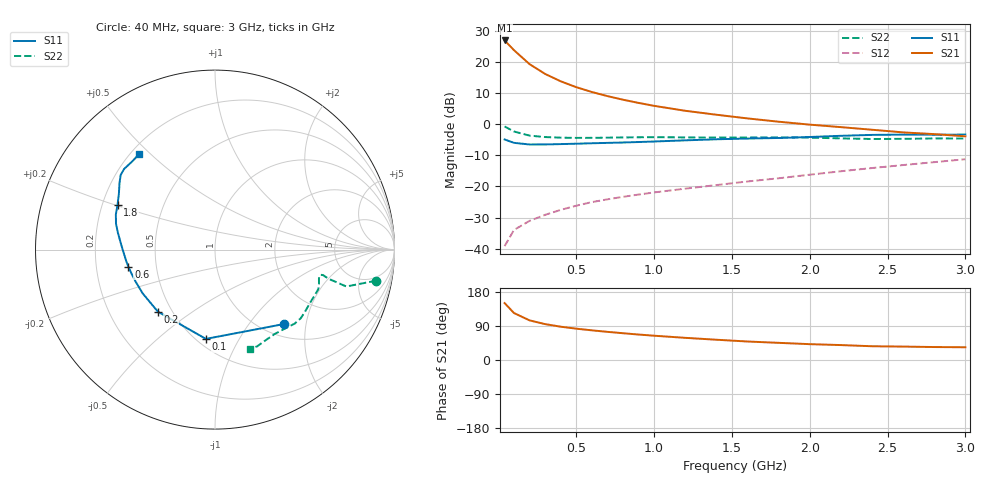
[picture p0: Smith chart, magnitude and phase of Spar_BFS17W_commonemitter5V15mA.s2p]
! Filename:  BFS17WD.S2P  Version:  4.0
! NXP part #: BFS17W  Date: Jun 1994
! Bias condition: Vce=5V, Ic=15mA
#  MHz  S  MA  R  50
! Freq  S11  S21  S12  S22  !GUM [dB]
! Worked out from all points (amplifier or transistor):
!   21 points, 40 MHz to 3 GHz, reference 50 ohm
!   highest |S21| = 26.8 dB at 40 MHz (marker M1)
!   |S21| within 3 dB of that: start of sweep to 97.95 MHz
!   unconditionally stable (mu >= 1): 325.1 MHz to 2.07 GHz
!   at 300 MHz: K = 0.98, MSG = 22.6 dB, |S12| = -29.1 dB
!   at 1 GHz: K = 1.20, MAG = 11.2 dB, |S12| = -21.9 dB
!   at 3 GHz: K = 0.95, MSG = 3.7 dB, |S12| = -11.3 dB
!   S11 on the Smith chart (normalised r, x): 40 MHz: 1.24, -1.51; 100 MHz: 0.56, -0.74; 200 MHz: 0.42, -0.37; 600 MHz: 0.34, -0.09; 1.8 GHz: 0.26, +0.21; 3 GHz: 0.23, +0.46
40  0.566 -47.1  21.93 150.2  0.011 71.1  0.915 -10.9
100  0.5 -95.8  15.33 124.0  0.02 58.8  0.76 -15.7
200  0.47 -132.6  9.156 104.6  0.028 57.9  0.653 -14.4
300  0.471 -148.7  6.371 94.7  0.035 59.9  0.619 -13.3
400  0.477 -158.0  4.854 87.9  0.042 62.8  0.605 -13.4
500  0.484 -164.0  3.905 82.7  0.049 65.0  0.6 -14.3
600  0.492 -168.9  3.27 78.3  0.056 66.8  0.601 -15.5
700  0.499 -172.9  2.809 74.3  0.062 68.3  0.605 -16.8
800  0.506 -176.6  2.46 70.7  0.068 69.9  0.61 -18.2
900  0.515 179.8  2.184 67.2  0.074 71.4  0.614 -19.6
1000  0.525 176.4  1.961 64.1  0.08 72.9  0.616 -21.1
1200  0.548 170.4  1.633 58.5  0.092 76.1  0.611 -24.6
1400  0.57 165.4  1.412 53.5  0.105 79.5  0.607 -29.3
1600  0.586 160.5  1.232 48.8  0.12 82.5  0.609 -34.4
1800  0.598 155.2  1.091 45.3  0.135 85.4  0.612 -38.7
2000  0.62 149.7  0.979 41.8  0.154 87.7  0.606 -42.9
2200  0.648 145.2  0.893 39.4  0.175 89.4  0.589 -48.0
2400  0.67 141.7  0.811 36.3  0.197 90.4  0.576 -54.6
2600  0.677 138.4  0.735 35.4  0.22 90.5  0.579 -61.3
2800  0.674 133.7  0.69 34.2  0.245 90.6  0.588 -66.5
3000  0.679 128.3  0.636 33.6  0.273 90.3  0.586 -70.7
